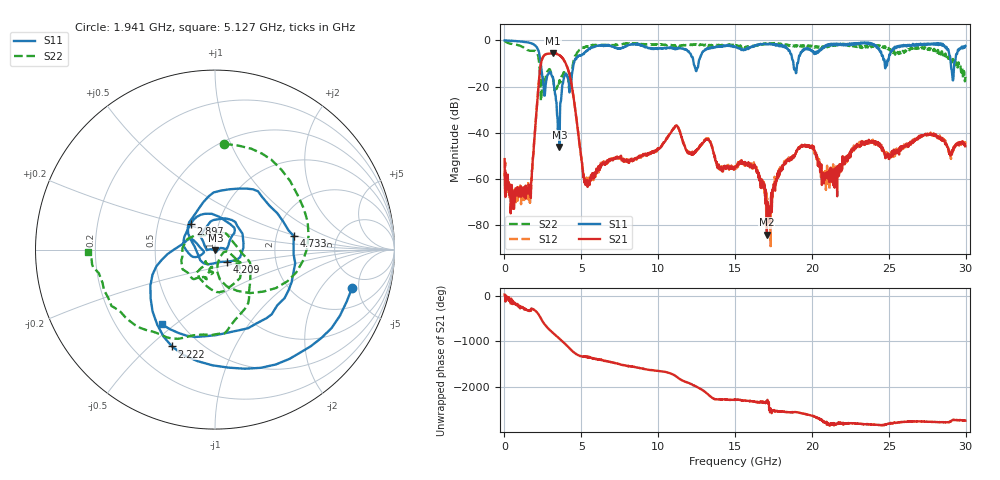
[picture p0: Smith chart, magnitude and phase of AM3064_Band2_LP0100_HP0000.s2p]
# Hz S DB R 50.0
!freq dBS11 angS11 dBS21 angS21 dBS12 angS12 dBS22 angS22
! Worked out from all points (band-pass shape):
!   1600 points, 10 MHz to 29.98 GHz, reference 50 ohm
!   highest |S21| = -5.49 dB at 3.159 GHz (marker M1); lowest = -84.2 dB at 17.07 GHz (marker M2)
!   |S21| within 3 dB of the highest: 2.43 GHz to 3.864 GHz (1.434 GHz wide, 45.6 % of centre)
!   lowest |S11| = -46.2 dB at 3.571 GHz (marker M3), VSWR 1.01, Z = 50.2 - j0.448 ohm
!   |S11| at or under -10 dB: 2.364 GHz to 4.506 GHz (2.142 GHz wide, 62.4 % of centre); 12.31 GHz to 12.62 GHz (307.9 MHz wide, 2.47 % of centre); 18.8 GHz to 19.05 GHz (251 MHz wide, 1.33 % of centre)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
!   |S22| runs from -26.3 to -0.2 dB; largest |S21 - S12| = 0.02
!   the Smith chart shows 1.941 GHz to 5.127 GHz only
!   S11 on the Smith chart (normalised r, x): 1.941 GHz: 3.61, -4.20; 2.222 GHz: 0.36, -0.59; 2.897 GHz: 0.73, +0.22; 4.209 GHz: 1.14, -0.15; 4.733 GHz: 2.49, +0.48; 5.127 GHz: 0.40, -0.45
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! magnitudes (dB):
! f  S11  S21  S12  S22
! 10 MHz  0.0  -51.5  -57.3  -0.2
! 1.584 GHz  -1.0  -62.5  -69.2  -4.4
! 1.941 GHz  -2.0  -43.4  -43.1  -4.6
! 2.222 GHz  -4.6  -19.3  -19.1  -7.9
! 2.897 GHz  -14.1  -5.7  -5.7  -12.5
! 3.159 GHz  -16.3  -5.5  -5.5  -16.6
! 3.571 GHz  -46.2  -6.5  -6.4  -17.4
! 4.209 GHz  -20.4  -14.3  -14.2  -21.2
! 4.733 GHz  -7.0  -36.7  -36.5  -5.2
! 5.015 GHz  -6.4  -51.9  -53.0  -3.7
! 5.127 GHz  -5.8  -59.2  -58.3  -3.0
! 10 GHz  -3.5  -47.1  -46.7  -1.8
! 11.18 GHz  -3.4  -36.9  -37.0  -2.5
! 15 GHz  -2.6  -55.3  -54.6  -2.0
! 16.28 GHz  -2.2  -54.5  -55.4  -2.3
! 17.07 GHz  -1.7  -84.2  -71.1  -1.6
! 19.99 GHz  -4.3  -46.5  -46.4  -2.3
! 20.8 GHz  -2.6  -58.7  -60.1  -2.6
! 23.36 GHz  -1.1  -44.6  -44.2  -3.1
! 25 GHz  -8.0  -49.6  -50.9  -3.3
! 29.18 GHz  -17.3  -48.0  -46.6  -8.0
! 29.98 GHz  -2.4  -45.9  -45.3  -15.8
